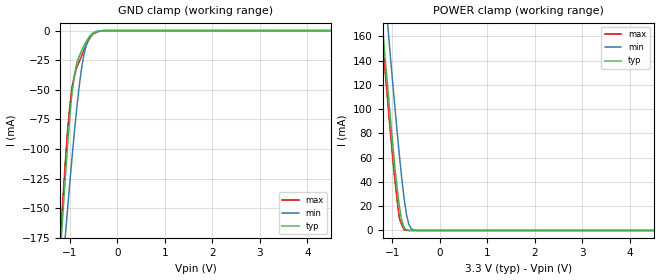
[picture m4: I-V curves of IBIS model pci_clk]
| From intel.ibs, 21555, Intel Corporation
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[Model]   pci_clk
Model_type   Input
Vinl = 0.99V
Vinh = 1.65V
|   typ   min   max
C_comp   4.000pF   2.000pF   6.000pF
[Voltage Range]   3.300V   3.135V   3.465V
[Temperature Range]   25.0   100.0   0.0
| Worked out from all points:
|   GND clamp passes 1 mA (typ) near -0.46 V on its own axis
|   POWER clamp passes 1 mA (typ) near -0.71 V on its own axis
[GND Clamp]
|   Voltage   I(typ)   I(min)   I(max)
-3.3V     -1.674A    -1.356A    -1.789A
-1.2V     -191mA     -227.1mA   -180.5mA
-1.15V    -159.4mA   -202.1mA   -147.1mA
-1.1V     -128.9mA   -177.6mA   -115.6mA
-1.05V    -100.2mA   -153.5mA   -87.26mA
-950mV    -52.01mA   -107.2mA   -47.88mA
-850mV    -27.3mA    -65.27mA   -30.97mA
-750mV    -17.19mA   -31.9mA    -21.66mA
-700mV    -12.93mA   -20.15mA   -16.67mA
-600mV    -5.942mA   -7.203mA   -8.052mA
-450mV    -906uA     -1.117mA   -1.7mA
6.55V     0A         0A         0A
[POWER Clamp]
|   Voltage   I(typ)   I(min)   I(max)
-3.3V     1.315A     1.34A      1.328A
-1.25V    192.8mA    244.5mA    178.6mA
-1.2V     167.3mA    220.4mA    155.6mA
-1.1V     121.2mA    173.1mA    109.1mA
-1.05V    98.12mA    149.4mA    86.03mA
-950mV    54.97mA    104.7mA    43.68mA
-850mV    19.85mA    62.7mA     10.07mA
-800mV    8.417mA    43.58mA    4.561mA
-750mV    2.519mA    26.64mA    513.5uA
-650mV    36.98uA    5.11mA     12.26uA
-500mV    365.5nA    94.16uA    9.304nA
6.55V     0A         0A         0A
